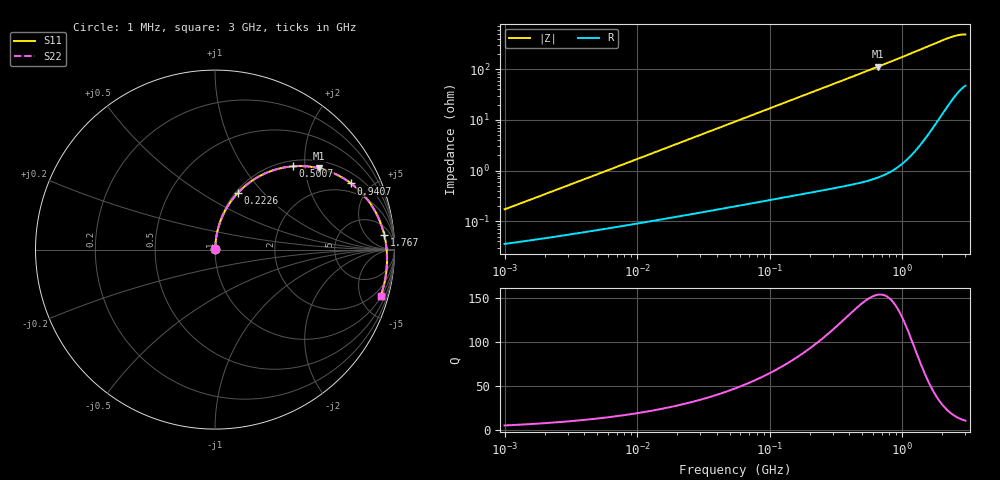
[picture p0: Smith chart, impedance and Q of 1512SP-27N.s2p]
# MHz  S  MA  R  50
!Freq  MagS11  AngS11  MagS21  AngS21  MagS12  AngS12  MagS22  AngS22
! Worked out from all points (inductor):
!   801 points, 1 MHz to 3 GHz, reference 50 ohm
!   read as one part in series: L = 26.9 nH near 1.041 MHz
!   highest Q = 154 at 656.1 MHz (marker M1), where L = 27.3 nH
!   S11 on the Smith chart (normalised r, x): 1 MHz: 1.00, +0.00; 222.6 MHz: 1.03, +0.74; 500.7 MHz: 1.11, +1.73; 940.7 MHz: 1.49, +3.80; 1.767 GHz: 11, +17; 3 GHz: 1.10, -7.09
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1  0.001672 77.5  0.9996 -0.1  0.9996 -0.1  0.001672 77.5
3.824029  0.006272 84.1  0.9994 -0.4  0.9994 -0.4  0.006272 84.1
14.47755  0.02364 86.0  0.9987 -1.4  0.9987 -1.4  0.02364 86.0
30.06344  0.04901 85.3  0.9973 -3.0  0.9973 -3.0  0.049 85.3
54.81117  0.08905 83.3  0.9941 -5.5  0.9941 -5.5  0.08903 83.3
82.62342  0.1335 80.8  0.9887 -8.2  0.9887 -8.2  0.1335 80.8
120.8637  0.1933 77.2  0.9783 -11.9  0.9783 -11.9  0.1933 77.2
161.5711  0.2547 73.5  0.9638 -15.8  0.9638 -15.8  0.2546 73.5
209.5995  0.3235 69.2  0.9428 -20.2  0.9428 -20.2  0.3233 69.2
222.5734  0.3412 68.0  0.9364 -21.4  0.9364 -21.4  0.3411 68.0
271.9047  0.4056 63.8  0.9102 -25.7  0.9102 -25.7  0.4054 63.8
332.1698  0.477 58.9  0.8749 -30.6  0.8749 -30.6  0.4767 58.9
413.9977  0.561 52.8  0.8236 -36.8  0.8236 -36.8  0.5606 52.8
500.7192  0.6348 47.0  0.7683 -42.6  0.7683 -42.6  0.6344 47.0
656.0968  0.7346 38.1  0.6739 -51.5  0.6739 -51.5  0.734 38.1
793.5315  0.7965 31.7  0.5997 -57.9  0.5997 -57.9  0.7957 31.7
940.7324  0.8437 25.9  0.531 -63.7  0.531 -63.7  0.8429 25.9
1295.912  0.9098 15.2  0.4051 -74.2  0.4051 -74.2  0.9089 15.2
1767.413  0.9471 4.8  0.2984 -83.7  0.2984 -83.7  0.9462 4.8
2095.27  0.9578 -1.0  0.2505 -88.7  0.2505 -88.7  0.9571 -1.0
2483.944  0.9623 -7.4  0.2141 -93.6  0.2141 -93.6  0.9619 -7.4
3000  0.9591 -15.7  0.1957 -99.8  0.1957 -99.8  0.9595 -15.7
